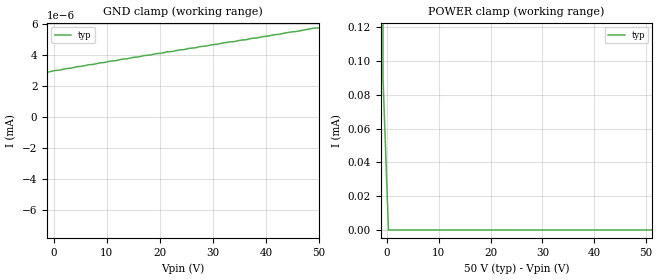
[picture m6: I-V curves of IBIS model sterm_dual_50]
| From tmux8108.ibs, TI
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| sterm_dual_50
[Model]   sterm_dual_50
Model_type   Terminator
|   typ   min   max
C_comp   4.014581e-12   NA   NA
[Voltage Range]   50   NA   NA
[Temperature Range]   27   NA   NA
[Power Clamp Reference]   50   NA   NA
[GND Clamp Reference]   0   NA   NA
[GND Clamp]
|   Voltage   I(typ)   I(min)   I(max)
-55V      -1.145A    NA         NA
-50.76V   -1.395mA   NA         NA
-49.7V    -674.8pA   NA         NA
-44.39V   -345.7pA   NA         NA
-34.85V   541.4pA    NA         NA
-26.36V   1.244nA    NA         NA
-13.64V   2.149nA    NA         NA
8.636V    3.506nA    NA         NA
50V       5.782nA    NA         NA
[POWER Clamp]
|   Voltage   I(typ)   I(min)   I(max)
-5V       744mA      NA         NA
-1.818V   145.4mA    NA         NA
-757.6mV  90.5uA     NA         NA
303mV     5.779nA    NA         NA
100V      -717.1pA   NA         NA
